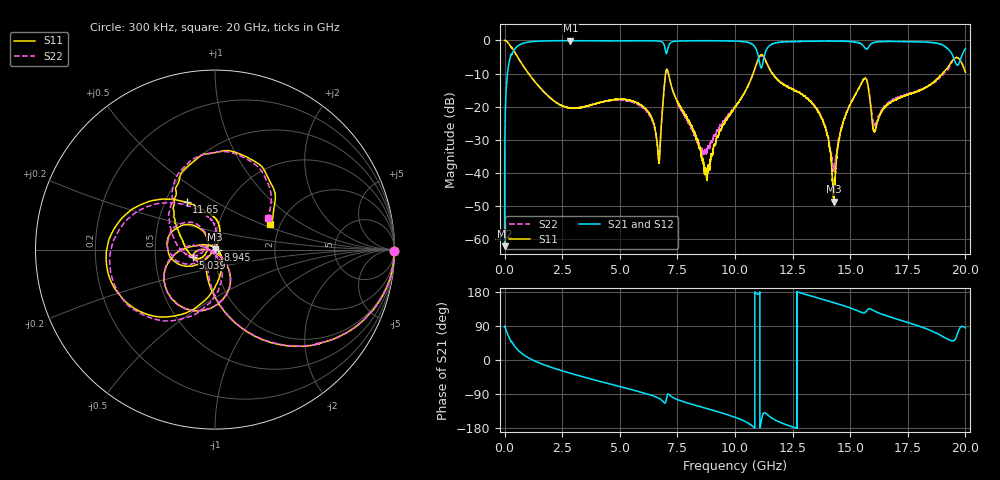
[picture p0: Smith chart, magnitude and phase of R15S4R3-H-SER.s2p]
!{R15S4R3}
!Johanson Technology Inc.
!www.johansontechnology.com
!Test Board Conditions:
!Substrate Type  RO4350B
!Substrate Thickness  20 mil
!Substrate Dk  3.66
!TL Type: GCPW
!TL Trace Width  34 mil
!TL Gap  10 mil
!Electrode orientation  Horizontal
!DUT TOPOLOGY	SERIES
!Mounting Pad LxW  26x52 mil
! Created Sat Feb  6 13:56:40 2021
# hz S ma R 50
! 2 Port Network Data from SP1.SP block
! freq  magS11  angS11  magS21  angS21  magS12  angS12  magS22  angS22
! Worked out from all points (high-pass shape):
!   20001 points, 300 kHz to 20 GHz, reference 50 ohm
!   highest |S21| = -0.06 dB at 2.855 GHz (marker M1); lowest = -62.1 dB at 300 kHz (marker M2)
!   |S21| within 3 dB of the highest: 393.6 MHz to 6.983 GHz (6.59 GHz wide, 179 % of centre); 11.35 GHz to 19.32 GHz (7.971 GHz wide, 52 % of centre)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
!   lowest |S11| = -48.6 dB at 14.29 GHz (marker M3), VSWR 1.01, Z = 49.7 + j0.264 ohm
!   |S11| at or under -10 dB: 1.044 GHz to 6.988 GHz (5.944 GHz wide, 148 % of centre); 7.113 GHz to 10.79 GHz (3.673 GHz wide, 41 % of centre); 11.62 GHz to 19 GHz (7.372 GHz wide, 48.2 % of centre)
!   |S22| runs from -39.4 to 0.0 dB; largest |S21 - S12| = 0.014
!   S11 on the Smith chart (normalised r, x): 300 kHz: open; 5.039 GHz: 0.78, -0.07; 8.945 GHz: 1.03, -0.01; 11.65 GHz: 0.64, +0.37; 20 GHz: 1.75, +0.54
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300000  1 -0.3  0.0007884 86.6  0.0007694 89.2  0.9981 -0.3
1.143e8  0.9546 -18.7  0.2943 71.1  0.2952 71.1  0.9534 -18.6
3.313e8  0.766 -43.9  0.6378 45.9  0.6393 45.9  0.7659 -43.7
1.0883e9  0.3016 -86.0  0.9512 3.9  0.9503 3.9  0.3006 -85.7
2.8553e9  0.095 -127.2  0.9931 -34.9  0.9922 -35.0  0.09623 -121.0
3.3343e9  0.0978 -134.7  0.9908 -43.2  0.9898 -43.2  0.09918 -129.9
5.0393e9  0.1302 -160.3  0.9856 -70.7  0.9855 -70.7  0.1263 -160.1
6.2213e9  0.0853 -179.8  0.9886 -90.4  0.9891 -90.3  0.08102 -178.6
6.6673e9  0.018 -153.1  0.9816 -100.2  0.9817 -100.2  0.01809 -144.8
7.0643e9  0.3627 -133.3  0.6908 -91.8  0.6908 -91.9  0.3642 -133.7
8.9453e9  0.01721 -10.1  0.9897 -131.0  0.9898 -131.1  0.02964 -92.6
1.00003e10  0.09805 -65.7  0.9781 -150.9  0.9788 -150.9  0.1008 -67.9
1.09723e10  0.4878 -129.7  0.6511 173.9  0.6556 174.0  0.477 -123.6
1.16493e10  0.308 120.9  0.8933 -155.2  0.8945 -155.3  0.3096 125.3
1.33343e10  0.1131 76.4  0.9747 168.4  0.9742 168.4  0.1162 88.4
1.42873e10  0.003708 134.4  0.9777 151.2  0.9797 151.3  0.01157 149.1
1.46533e10  0.05184 -132.7  0.9727 144.5  0.9746 144.4  0.05158 -137.6
1.55533e10  0.2515 -169.9  0.8428 124.4  0.8471 123.9  0.2479 -174.4
1.60493e10  0.04277 171.5  0.9396 129.2  0.9391 129.3  0.05308 154.8
1.66673e10  0.1115 -153.7  0.9694 114.9  0.9611 114.8  0.1146 -161.9
1.90993e10  0.3451 131.1  0.8156 59.1  0.8165 59.1  0.3293 140.7
2e10  0.3303 24.8  0.7506 84.7  0.7482 85.0  0.34 30.4
